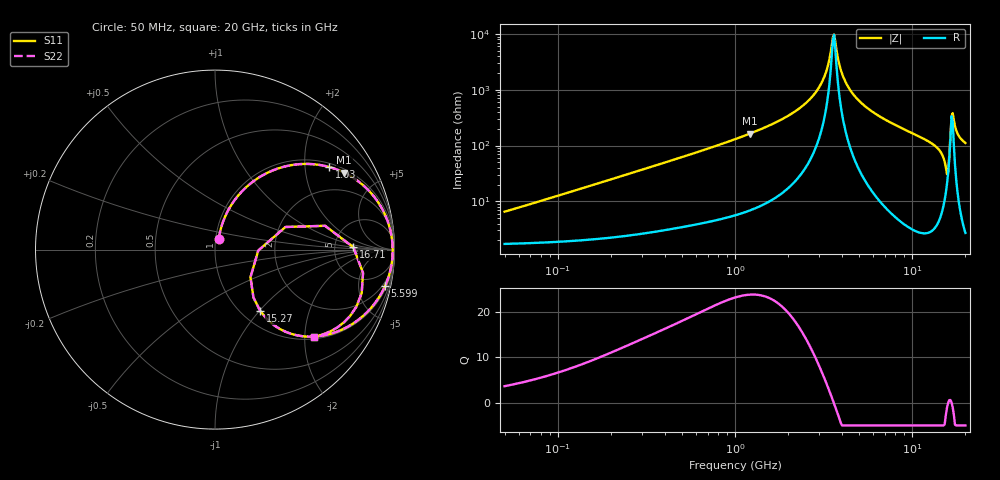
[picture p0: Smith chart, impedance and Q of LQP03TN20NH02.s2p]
!Murata Part Number: LQP03TN20NH02
!These Parameters are Measured in Series Mode Connection
!  o--[Z]--o
!Port1  Port2
!  o-------o
!Freq. Start=50[MHz] Stop=20[GHz], 401[Steps]
# Hz S RI R 50
!Freq.(Hz) S11(Real) S11(Imag) S21(Real) S21(Imag) S12(Real) S12(Imag) S22(Real) S22(Imag)
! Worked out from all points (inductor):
!   401 points, 50 MHz to 20 GHz, reference 50 ohm
!   read as one part in series: L = 19.9 nH near 51.52 MHz
!   highest Q = 23.8 at 1.215 GHz (marker M1), where L = 21.4 nH
!   self-resonance near 3.572 GHz
!   S11 on the Smith chart (normalised r, x): 50 MHz: 1.03, +0.13; 1.03 GHz: 1.12, +2.68; 5.599 GHz: 1.40, -9.35; 15.27 GHz: 1.21, -1.01; 16.71 GHz: 7.71, +0.50; 20 GHz: 1.05, -2.23
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5e7  0.0207 0.0605  0.9793 -0.0605  0.9793 -0.0605  0.0207 0.0605
1.364002e8  0.0459 0.1584  0.9541 -0.1584  0.9541 -0.1584  0.0459 0.1584
3.721004e8  0.1891 0.361  0.8109 -0.361  0.8109 -0.361  0.1891 0.361
1e9  0.6222 0.4637  0.3778 -0.4637  0.3778 -0.4637  0.6222 0.4637
1.030411e9  0.6377 0.4597  0.3623 -0.4597  0.3623 -0.4597  0.6377 0.4597
1.214974e9  0.72 0.4285  0.28 -0.4285  0.28 -0.4285  0.72 0.4285
1.99176e9  0.9094 0.263  0.0906 -0.263  0.0906 -0.263  0.9094 0.263
2.728004e9  0.9718 0.1274  0.0282 -0.1274  0.0282 -0.1274  0.9718 0.1274
3.168813e9  0.9858 0.0598  0.0142 -0.0598  0.0142 -0.0598  0.9858 0.0598
3.626126e9  0.9901 -0.00179  0.00994 0.00179  0.00994 0.00179  0.9901 -0.00179
3.967106e9  0.9885 -0.0431  0.0115 0.0431  0.0115 0.0431  0.9885 -0.0431
4.212059e9  0.9855 -0.0706  0.0145 0.0706  0.0145 0.0706  0.9855 -0.0706
5.598765e9  0.9485 -0.2008  0.0515 0.2008  0.0515 0.2008  0.9485 -0.2008
7.442007e9  0.8695 -0.3248  0.1305 0.3248  0.1305 0.3248  0.8695 -0.3248
1.314879e10  0.5223 -0.485  0.4777 0.485  0.4777 0.485  0.5223 -0.485
1.460232e10  0.3633 -0.4434  0.6367 0.4434  0.6367 0.4434  0.3633 -0.4434
1.527346e10  0.2513 -0.3415  0.7487 0.3415  0.7487 0.3415  0.2513 -0.3415
1.597544e10  0.2412 -0.00494  0.7588 0.00494  0.7588 0.00494  0.2412 -0.00494
1.670968e10  0.7711 0.013  0.2289 -0.013  0.2289 -0.013  0.7711 0.013
1.721783e10  0.8173 -0.2425  0.1827 0.2425  0.1827 0.2425  0.8173 -0.2425
1.800918e10  0.7179 -0.4056  0.2821 0.4056  0.2821 0.4056  0.7179 -0.4056
2e10  0.5522 -0.4853  0.4478 0.4853  0.4478 0.4853  0.5522 -0.4853
